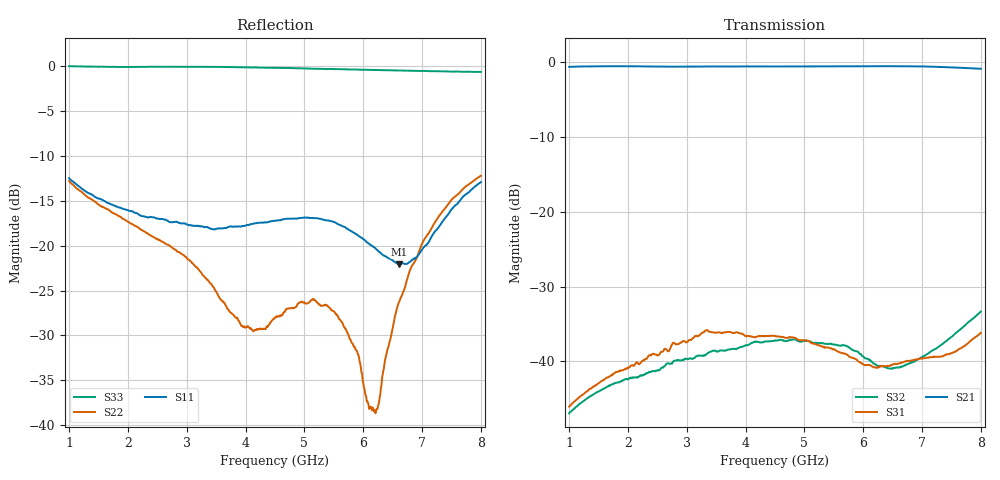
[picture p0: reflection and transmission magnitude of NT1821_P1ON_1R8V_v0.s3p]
! NT1821 PC-P1 ON state
! Port1:PC, Port2:P1, Port3:P2
! VDD=1.8V, VCTL=1.2V
# hz S ma R 50
! 3 Port Network Data from SP1.SP block
! freq  magS11  angS11  magS12  angS12  magS13  angS13
!  magS21  angS21
!  magS22  angS22  magS23  angS23
!  magS31  angS31  magS32  angS32
!  magS33  angS33
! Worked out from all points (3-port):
!   701 points, 1 GHz to 8 GHz, reference 50 ohm
!   strongest paths, dB at 1 GHz, 2.75 GHz, 4.5 GHz, 6.25 GHz, 8 GHz:
!     S21: -0.7, -0.6, -0.6, -0.6, -0.9
!     S31: -46.0, -37.8, -36.6, -40.8, -36.2
!     S32: -46.9, -40.3, -37.3, -40.6, -33.3
!   lowest |S11| = -22.1 dB at 6.61 GHz (marker M1), VSWR 1.17, Z = 47.7 - j7.38 ohm
!   |S11| at or under -10 dB: start of sweep to end of sweep
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1e9  0.2382 -76.6  0.9291 1.7  0.004985 75.8
     0.9274 1.7  0.2298 -76.9  0.004499 71.8
     0.004989 75.5  0.004496 71.7  1.003 -14.1
3.33e9  0.1272 -57.9  0.9335 -28.2  0.01612 62.6
        0.9327 -28.3  0.06551 -116.8  0.0111 64.1
        0.0161 62.2  0.0111 63.7  0.9943 -39.0
3.96e9  0.1286 -44.8  0.9345 -34.6  0.01519 51.3
        0.9334 -34.6  0.03525 -167.5  0.01262 61.9
        0.01513 51.1  0.01261 61.2  0.989 -45.9
4.5e9  0.1378 -38.3  0.9343 -40.3  0.01482 50.2
       0.9329 -40.3  0.03965 131.9  0.01375 56.2
       0.01475 49.7  0.01371 55.6  0.9817 -54.0
5.5e9  0.1359 -44.2  0.9364 -50.4  0.0121 47.0
       0.9348 -50.1  0.04308 94.9  0.013 50.7
       0.01208 46.3  0.01295 49.9  0.9674 -75.1
5.89e9  0.1157 -54.1  0.937 -54.3  0.01026 50.8
        0.9356 -54.3  0.02592 102.6  0.01159 49.6
        0.01027 50.0  0.01167 48.6  0.96 -85.0
6.2e9  0.09724 -68.3  0.9377 -57.7  0.009145 62.7
       0.9363 -57.7  0.01184 177.8  0.009541 56.2
       0.00915 61.9  0.009557 55.5  0.955 -93.0
6.61e9  0.07887 -103.0  0.9384 -62.4  0.009692 77.4
        0.9372 -62.3  0.04854 -127.7  0.009076 76.8
        0.009702 76.4  0.009075 75.6  0.9497 -102.7
7.25e9  0.1231 -164.2  0.9289 -69.8  0.01069 92.5
        0.9274 -70.0  0.1403 -125.9  0.01225 101.7
        0.01073 91.9  0.01223 101.2  0.9395 -114.7
8e9  0.2265 168.5  0.9023 -78.3  0.01554 116.9
     0.9008 -78.3  0.2458 -128.1  0.02145 114.1
     0.01551 116.4  0.02151 113.6  0.9308 -123.0
